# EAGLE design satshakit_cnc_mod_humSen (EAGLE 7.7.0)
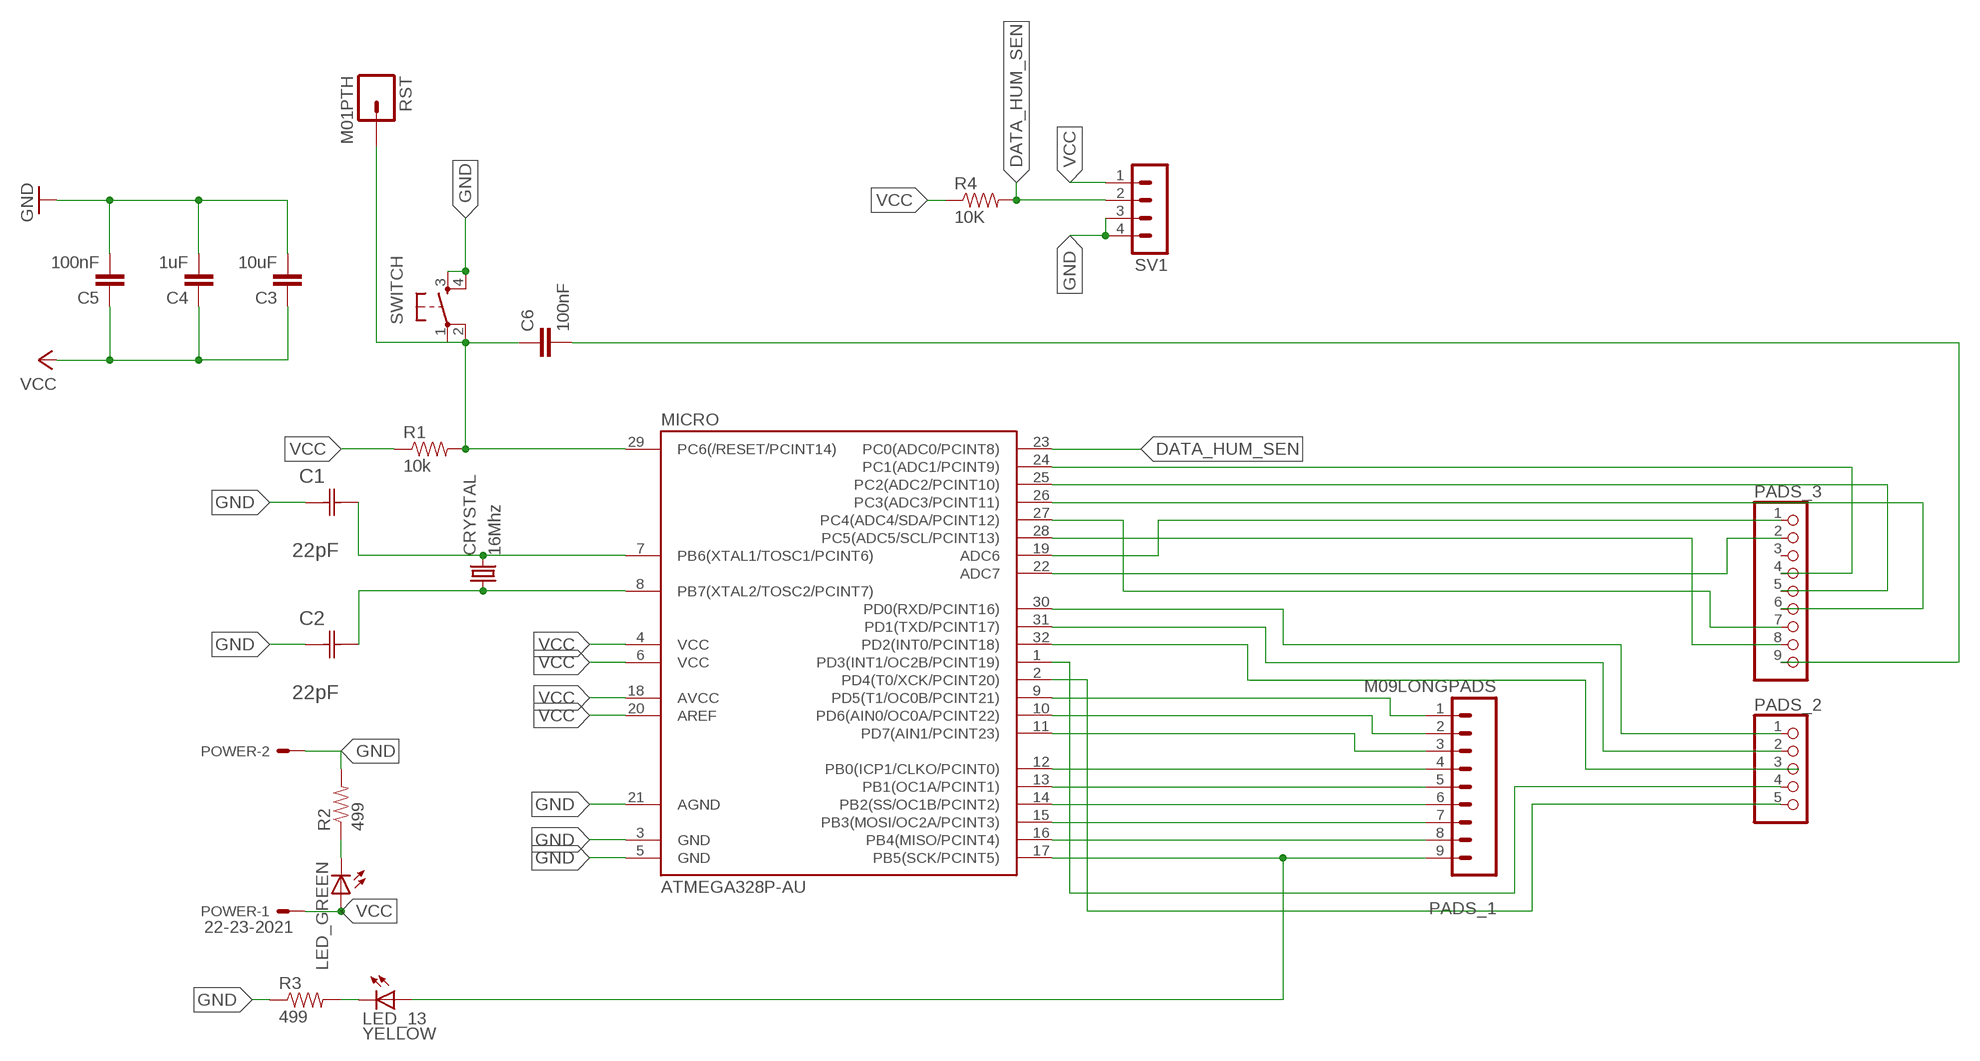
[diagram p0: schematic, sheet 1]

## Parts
C1  22pF  0612ZC225MAT2A  [CAPC3216X178N]
C2  22pF  0612ZC225MAT2A  [CAPC3216X178N]
C3  10uF  CAP1206  [1206]
C4  1uF  CAP1206  [1206]
C5  100nF  CAP1206  [1206]
C6  100nF  CAP1206  [1206]
CRYSTAL  16Mhz  CSM-7X-DU  [CSM-7X-DU]
LED_13  YELLOW  LED1206  [1206]
LED_GREEN  LED1206  [1206]
MICRO  ATMEGA328P-AU  ATMEGA48/88/168-AU  [TQFP32-08]
PADS_1  M09LONGPADS  [1X09_LONGPADS]
PADS_2  PINHD-1X5  [1X05]
PADS_3  PINHD-1X9  [1X09]
POWER  22-23-2021  [22-23-2021]
R1  10k  RESISTOR1206  [1206]
R2  499  RESISTOR1206  [1206]
R3  499  RESISTOR1206  [1206]
R4  10K  RESISTOR1206  [1206]
RST  M01PTH  [1X01]
SV1  MA04-1  [MA04-1]
SWITCH  6MM_SWITCH6MM_SWITCH  [6MM_SWITCH]

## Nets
DATA_HUM_SEN: MICRO.23(PC0(ADC0/PCINT8)) R4.2 SV1.2
GND: C1.1(C1) C2.1(C1) C3.2 C4.2 C5.2 MICRO.3(GND) MICRO.5(GND) MICRO.21(AGND) POWER.2 R2.2 R3.1 SV1.3 SV1.4 SWITCH.3(S) SWITCH.4(S1)
N$1: MICRO.9(PD5(T1/OC0B/PCINT21)) PADS_1.1
N$2: C1.2(C2) CRYSTAL.2 MICRO.7(PB6(XTAL1/TOSC1/PCINT6))
N$3: C6.2 PADS_3.9
N$4: MICRO.10(PD6(AIN0/OC0A/PCINT22)) PADS_1.2
N$5: MICRO.11(PD7(AIN1/PCINT23)) PADS_1.3
N$6: MICRO.12(PB0(ICP1/CLKO/PCINT0)) PADS_1.4
N$7: MICRO.13(PB1(OC1A/PCINT1)) PADS_1.5
N$8: MICRO.14(PB2(SS/OC1B/PCINT2)) PADS_1.6
N$9: C2.2(C2) CRYSTAL.1 MICRO.8(PB7(XTAL2/TOSC2/PCINT7))
N$10: MICRO.15(PB3(MOSI/OC2A/PCINT3)) PADS_1.7
N$11: MICRO.16(PB4(MISO/PCINT4)) PADS_1.8
N$12: LED_13.1(A) MICRO.17(PB5(SCK/PCINT5)) PADS_1.9
N$13: MICRO.19(ADC6) PADS_3.1
N$14: MICRO.22(ADC7) PADS_3.2
N$16: MICRO.24(PC1(ADC1/PCINT9)) PADS_3.4
N$17: MICRO.25(PC2(ADC2/PCINT10)) PADS_3.5
N$18: MICRO.26(PC3(ADC3/PCINT11)) PADS_3.6
N$19: MICRO.27(PC4(ADC4/SDA/PCINT12)) PADS_3.7
N$20: MICRO.30(PD0(RXD/PCINT16)) PADS_2.1
N$21: MICRO.31(PD1(TXD/PCINT17)) PADS_2.2
N$22: MICRO.32(PD2(INT0/PCINT18)) PADS_2.3
N$23: MICRO.1(PD3(INT1/OC2B/PCINT19)) PADS_2.4
N$24: MICRO.2(PD4(T0/XCK/PCINT20)) PADS_2.5
N$25: MICRO.28(PC5(ADC5/SCL/PCINT13)) PADS_3.8
N$26: LED_GREEN.2(C) R2.1
N$27: LED_13.2(C) R3.2
N$28: C6.1 MICRO.29(PC6(/RESET/PCINT14)) R1.2 RST.1 SWITCH.1(P) SWITCH.2(P1)
VCC: C3.1 C4.1 C5.1 LED_GREEN.1(A) MICRO.4(VCC) MICRO.6(VCC) MICRO.18(AVCC) MICRO.20(AREF) POWER.1 R1.1 R4.1 SV1.1
Unconnected: PADS_3.3

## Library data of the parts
C1 C2 = AVX_By_element14_Batch_1:0612ZC225MAT2A: Capacitor 1206; MPN: 0612ZC225MAT2A; OC_FARNELL: -; OC_NEWARK: 12N3209; SUPPLIER: AVX; TOLERANCE: ±20%; VALUE: 2.2µF; VOLTAGERATING: 10V
C3-C6 = 01_SparkFun:CAP: Capacitor
CRYSTAL = 01_FAB_Hello:CSM-7X-DU: SMD CRYSTAL; OC_FARNELL: unknown; OC_NEWARK: unknown
LED_13 LED_GREEN = 01_FAB_Hello:LED
MICRO = atmega8:ATMEGA48/88/168
PADS_1 = 01_SparkFun:M09: Header 9 Standard 9-pin 0.1" header. Use with straight break away headers (SKU : PRT-00116), right angle break away headers (PRT-00553), swiss pins (PRT-00743), machine pins (PRT-00117), and female headers (PRT-00115).
PADS_2 = pinhead:PINHD-1X5: PIN HEADER
PADS_3 = pinhead:PINHD-1X9: PIN HEADER
POWER = con-molex:22-23-2021: .100" (2.54mm) Center Header - 2 Pin; MF: MOLEX; MPN: 22-23-2021; OC_FARNELL: 1462926; OC_NEWARK: 25C3832
R1-R4 = 01_SparkFun:RESISTOR: Resistor
RST = 01_SparkFun:M01: Header 1
SV1 = con-lstb:MA04-1: PIN HEADER; OC_FARNELL: unknown; OC_NEWARK: unknown
SWITCH = 01_FAB_Hello:6MM_SWITCH: OMRON SWITCH

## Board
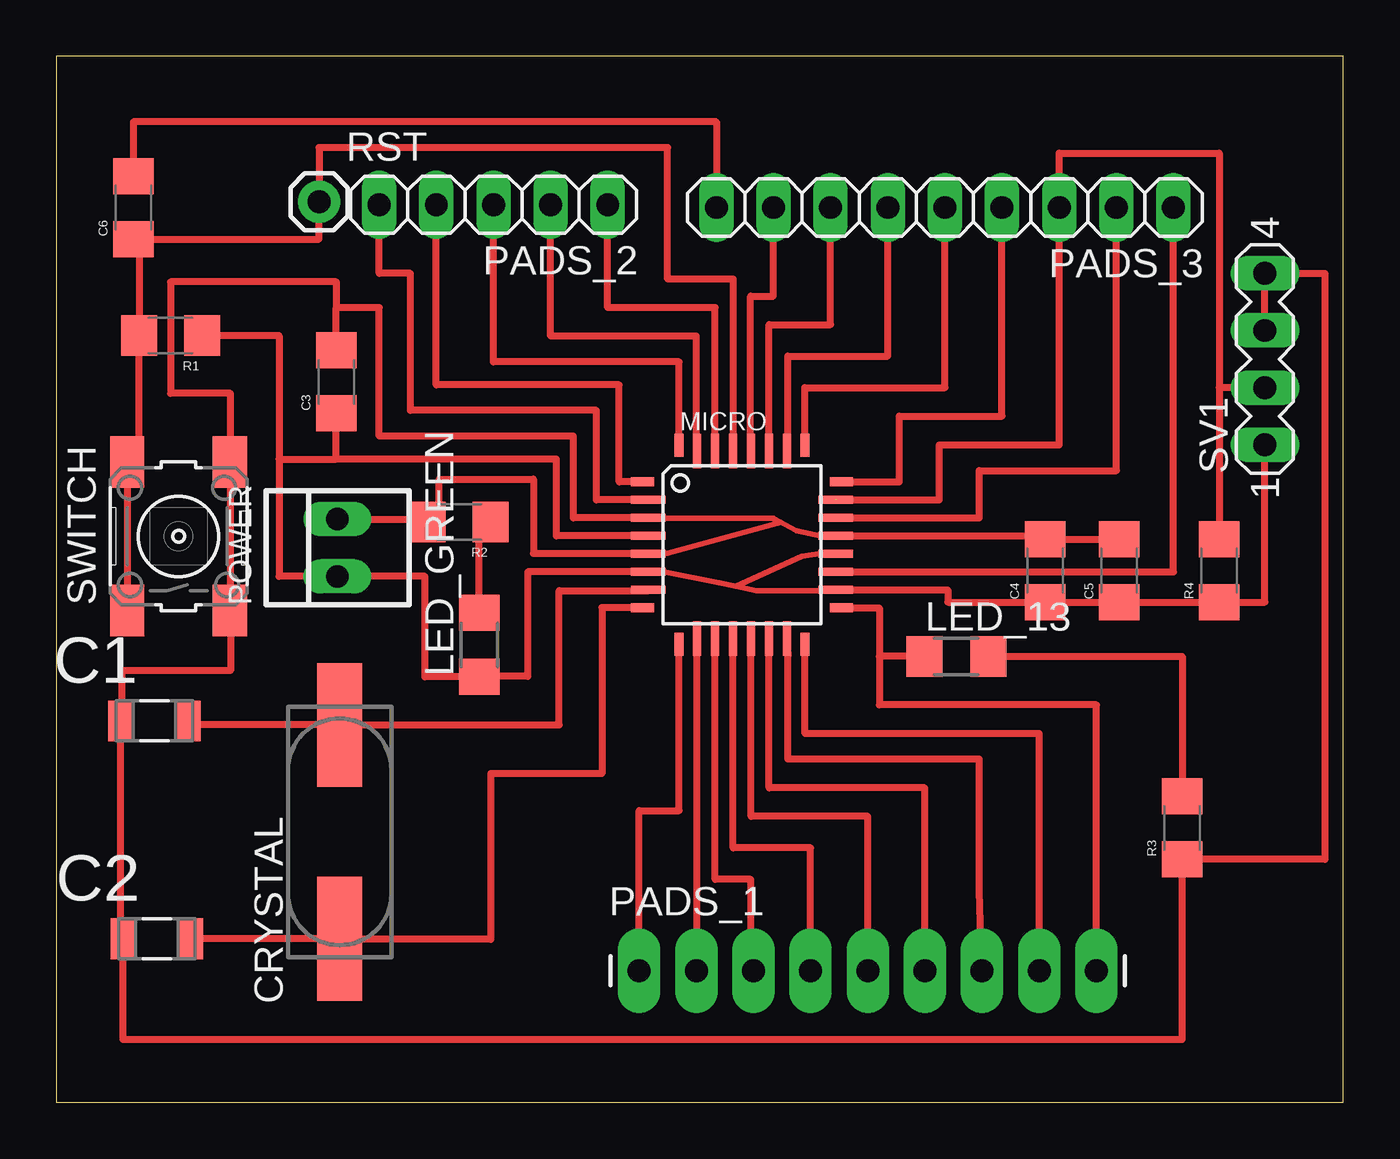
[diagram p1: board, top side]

Size 57.2 x 46.47 mm. Coordinates in mm from the lower left corner, seen from the top.
Outline: 0,0 57.2,0 57.2,46.47 0,46.47 0,0
Copper layers (1*16): Top 0.035mm / dielectric 1.5mm / Bottom 0.035mm
Design rules "default": minimum track width 10mil, minimum drill 24mil, track to track 8mil, track to pad 8mil, pad to pad 8mil, via to via 8mil, smd to smd 8mil, copper to edge 40mil, drill to drill 8mil, minimum pad ring 10mil, minimum via ring 8mil, stop-mask expansion 4mil, vias tented up to drill 0mil, thermal gap 10mil

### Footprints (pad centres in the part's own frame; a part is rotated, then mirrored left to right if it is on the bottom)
CAPC3216X178N = smd 1.118 x 1.803: 1 -1.499,0; 2 1.499,0
1206 = smd 1.6 x 1.8: 1 -1.4,0; 2 1.4,0
CSM-7X-DU = smd 5.5 x 2: 1 -4.75,0; 2 4.75,0
1206' = smd 1.6 x 1.803: 1 -1.422,0; 2 1.422,0
TQFP32-08 = smd 1.016 x 0.406: 1 -4.42,2.8; 8 -4.42,-2.8; 17 4.42,-2.8; 24 4.42,2.8 | smd 1.524 x 0.356: 2 -4.166,2; 3 -4.166,1.2; 4 -4.166,0.4; 5 -4.166,-0.4; 6 -4.166,-1.2; 7 -4.166,-2; 18 4.166,-2; 19 4.166,-1.2; 20 4.166,-0.4; 21 4.166,0.4; 22 4.166,1.2; 23 4.166,2 | smd 0.406 x 1.016: 9 -2.8,-4.42; 16 2.8,-4.42; 25 2.8,4.42; 32 -2.8,4.42 | smd 0.356 x 1.524: 10 -2,-4.166; 11 -1.2,-4.166; 12 -0.4,-4.166; 13 0.4,-4.166; 14 1.2,-4.166; 15 2,-4.166; 26 2,4.166; 27 1.2,4.166; 28 0.4,4.166; 29 -0.4,4.166; 30 -1.2,4.166; 31 -2,4.166
1X09_LONGPADS = drill 1.016 pad 1.88 long: 1 0,0; 2 2.54,0; 3 5.08,0; 4 7.62,0; 5 10.16,0; 6 12.7,0; 7 15.24,0; 8 17.78,0; 9 20.32,0
1X05 = drill 1.016 long: 1 -5.08,0; 2 -2.54,0; 3 0,0; 4 2.54,0; 5 5.08,0
1X09 = drill 1.016 long: 1 -10.16,0; 2 -7.62,0; 3 -5.08,0; 4 -2.54,0; 5 0,0; 6 2.54,0; 7 5.08,0; 8 7.62,0; 9 10.16,0
22-23-2021 = drill 1 long: 1 -1.27,0; 2 1.27,0
1X01 = drill 1.016 pad 1.88: 1 0,0
MA04-1 = drill 1.016 long: 1 -3.81,0; 2 -1.27,0; 3 1.27,0; 4 3.81,0
6MM_SWITCH = smd 2.286 x 1.524: 1 -3.302,2.286; 2 3.302,2.286; 3 -3.302,-2.286; 4 3.302,-2.286

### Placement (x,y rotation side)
C1  4.37,16.94 0 top
C2  4.47,7.26 0 top
C3  12.45,32 90 top
C4  43.94,23.62 90 top
C5  47.24,23.62 90 top
C6  3.43,39.75 90 top
CRYSTAL  12.6,12.01 90 top
LED_13  YELLOW  [1206']  40.01,19.81 0 top
LED_GREEN  [1206']  18.8,20.32 90 top
MICRO  30.48,24.77 0 top
PADS_1  25.91,5.84 0 top
PADS_2  19.43,39.88 180 top
PADS_3  39.5,39.75 180 top
POWER  12.5,24.64 90 top
R1  5.08,34.06 180 top
R2  17.91,25.78 180 top
R3  50.04,12.19 90 top
R4  51.69,23.62 90 top
RST  11.68,40.01 0 top
SV1  53.72,33.02 90 top
SWITCH  5.44,25.15 90 top

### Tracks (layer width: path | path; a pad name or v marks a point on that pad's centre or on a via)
DATA_HUM_SEN  (1 unrouted)
  Top 0.305: SV1.2 51.69,31.75 | 51.69,31.75 R4.2 | MICRO.23 39.24,26.77 39.24,29.21 44.58,29.21 44.58,42.16 51.69,42.16 51.69,31.75
GND
  Top 0.254: MICRO.3 26.34,25.94 31.87,25.94 | 31.87,25.94 32.89,25.4 34.04,25.15 | 26.92,24.38 27.18,24.38 32.05,25.73 | 32.05,25.73 32.19,25.77 | 31.87,25.94 32.05,25.73
  Top 0.305: MICRO.5 | MICRO.21 | C1.1 2.87,7.26 C2.1 2.97,2.79 50.04,2.79 R3.1 56.39,10.79 56.39,36.83 SV1.4 SV1.3 | C1.1 2.79,16.94 | MICRO.5 26.31,24.38 21.21,24.38 21.21,27.69 17.02,27.69 17.02,25.65 R2.2 17.02,25.91 POWER.2 | C1.1 2.92,16.94 2.92,19.18 7.75,19.18 7.75,21.84 | MICRO.21 43.94,25.16 C4.2 C5.2 | 26.92,24.38 MICRO.5 | MICRO.21 34.04,25.15 | MICRO.3 22.99,25.96 22.99,29.59 14.35,29.59 14.35,35.31 12.45,35.31 | C3.2 12.45,35.31 | SWITCH.3 7.75,21.84 | 7.75,21.84 7.75,27.81 7.72,27.81 SWITCH.4 7.75,28.45 7.75,31.5 5.08,31.5 5.08,36.45 12.45,36.45 12.45,35.31
N$1
  Top 0.305: PADS_1.1 25.91,12.95 27.68,12.95 MICRO.9
N$2
  Top 0.305: 5.87,16.76 C1.2 5.87,16.76 | MICRO.7 26.31,22.73 22.35,22.73 22.35,16.76 CRYSTAL.2 5.87,16.76
N$3
  Top 0.305: PADS_3.9 29.34,43.56 3.43,43.56 C6.2
N$4
  Top 0.305: PADS_1.2 28.48,9.4 MICRO.10
N$5
  Top 0.305: MICRO.11 29.28,9.91 30.86,9.91 30.86,6.48 30.99,6.48 PADS_1.3
N$6
  Top 0.305: 30.1,20.6 MICRO.12 30.08,11.3 33.53,11.3 PADS_1.4
N$7
  Top 0.305: PADS_1.5 36.07,12.7 30.88,12.7 MICRO.13
N$8
  Top 0.305: PADS_1.6 38.61,13.97 31.68,13.97 MICRO.14
N$9
  Top 0.305: 5.97,7.24 C2.2 | MICRO.8 24.26,21.97 24.26,14.61 19.3,14.61 19.3,7.24 12.6,7.24 CRYSTAL.1 C2.2 | C2.2
N$10
  Top 0.305: PADS_1.7 41.02,9.4 41.02,15.24 32.51,15.24 32.51,19.81 MICRO.15
N$11
  Top 0.305: MICRO.16 33.28,16.38 43.69,16.38 PADS_1.8
N$12
  Top 0.305: PADS_1.9 46.23,17.65 36.58,17.65 36.58,19.81 | LED_13.1 36.58,19.81 | MICRO.17 36.58,21.96 36.58,19.81
N$13
  Top 0.305: MICRO.19 49.66,23.57 PADS_3.1
N$14
  Top 0.305: MICRO.22 41.02,25.96 41.02,28.07 47.12,28.07 PADS_3.2
N$16
  Top 0.305: MICRO.24 37.47,27.57 37.47,30.48 42.04,30.48 PADS_3.4
N$17
  Top 0.305: MICRO.25 33.27,31.75 39.5,31.75 PADS_3.5
N$18
  Top 0.305: MICRO.26 32.51,28.93 32.51,33.15 36.96,33.15 PADS_3.6
N$19
  Top 0.305: MICRO.27 31.68,34.54 34.42,34.54 PADS_3.7
N$20
  Top 0.305: PADS_2.1 24.51,35.31 29.28,35.31 MICRO.30
N$21
  Top 0.305: MICRO.31 28.45,28.93 28.45,34.04 21.97,34.04 PADS_2.2
N$22
  Top 0.305: MICRO.32 27.69,32.89 19.43,32.89 PADS_2.3
N$23
  Top 0.305: MICRO.1 25.02,27.57 25.02,31.88 16.89,31.88 PADS_2.4
N$24
  Top 0.305: MICRO.2 24,26.77 24,30.73 15.75,30.73 15.75,36.83 14.35,36.83 PADS_2.5
N$25
  Top 0.305: MICRO.28 30.86,28.93 30.86,35.81 31.88,35.81 PADS_3.8
N$26
  Top 0.305: 19.69,25.53 R2.1 19.31,25.4 18.8,25.4 LED_GREEN.2
N$27
  Top 0.305: LED_13.2 50.04,19.81 R3.2
N$28
  Top 0.305: MICRO.29 30.1,28.93 30.1,36.58 27.18,36.58 27.18,42.42 11.68,42.42 RST.1 11.68,38.35 3.68,38.35 | R1.2 3.43,34.06 | R1.2 3.68,28.45 SWITCH.2 SWITCH.1 | C6.1 3.68,38.35 | 3.68,38.35 R1.2
VCC
  Top 0.254: 27,23.57 29.45,23.07 30.21,22.92 | 30.21,22.92 31.12,22.73 34.65,22.73 | MICRO.20 34.04,24.37 34.04,24.38 33.15,24.26 30.21,22.92
  Top 0.305: MICRO.18 | MICRO.20 34.04,24.38 | MICRO.4 22.23,25.16 22.23,28.57 12.45,28.57 | 9.91,28.57 9.91,34.06 R1.1 | 9.91,28.57 9.91,23.37 POWER.1 16.38,23.37 16.38,18.9 LED_GREEN.1 18.8,18.92 20.95,18.92 20.95,23.57 MICRO.6 27,23.57 | 34.65,22.73 MICRO.18 | MICRO.18 39.62,22.77 39.62,22.23 C4.1 C5.1 R4.1 53.72,22.22 SV1.1 | 9.91,28.57 12.45,28.57 | 12.45,28.57 C3.1 12.83,30.6 12.83,30.35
